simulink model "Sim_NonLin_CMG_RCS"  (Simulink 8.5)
settings: Solver=ode45  StartTime=0.0  StopTime=3600  FixedStep=Ts*2  RelTol=1e-3
InitFcn:
  | start3
StopFcn:
  | Pl
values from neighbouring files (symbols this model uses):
  Ave = [    [vehicle_flex34.m]    (also in vehicle_rigid.m)
  Bve = [    [vehicle_flex34.m]    (also in vehicle_rigid.m)
  CB2L = [cpsi, -cphi*spsi,  sphi*spsi;          0,    cphi,      -sphi;          0,    sphi*cpsi,  cphi*cpsi]/cpsi    [Rigbod_Dynam_LVLH.m]    (also in start.m = eye(3); start2.m = eye(3); start3.m = eye(3); start1.m = eye(3))
  com_dir = com_dir/sqrt(com_dir'*com_dir)    [start.m]    (also in start2.m; start3.m; start1.m)
  Cve = [    [vehicle_flex34.m]    (also in vehicle_rigid.m)
  d2r = pi/180    (= 0.0174532925199)    [start.m]    (also in start2.m; start3.m; Dead_Band_DF.m; start1.m)
  Dve = [    [vehicle_flex34.m]    (also in vehicle_rigid.m)
  ini = [wbo; atto; Hco]    [start.m]    (also in start2.m; start3.m; start1.m)
  J = [0.119416e9, -0.476e7,   -0.1216e7;     -0.476e7,     0.40408e8, -0.30121e6;     -0.1216e7,   -0.30121e6,  0.110166e9]    [start.m]    (also in start2.m; start3.m; start1.m)
  KshC = 2*Wdot_Lim_CMG/WlimC    [start.m]    (also in start2.m; start3.m; start1.m)
  KshR = 2*Wdot_Lim_RCS/WlimR    [start.m]    (also in start2.m; start3.m; start1.m)
  nt = 12    [start.m]    (also in start2.m; start3.m; start1.m)
  omg = 20*wo    (= 0.022)    [start.m]    (also in start2.m; start3.m; start1.m)
  r2d = 180/pi    (= 57.2957795131)    [start.m]    (also in start2.m; start3.m; start1.m)
  thecmd = 20    [start.m]    (also in start2.m; start3.m; start1.m = 0.1)
  Wdot_Lim_CMG = 0.0001*d2r    (= 1.74532925199e-06)    [start.m]    (also in start2.m; start3.m; start1.m)
  Wdot_Lim_RCS = 0.02*d2r    (= 0.000349065850399)    [start.m]    (also in start2.m; start3.m; start1.m)
  Wlim_CMG = 0.01*d2r    (= 0.000174532925199)    [start.m]    (also in start2.m; start3.m; start1.m)
  Wlim_RCS = 0.6*d2r    (= 0.010471975512)    [start.m]    (also in start2.m; start3.m; start1.m)
  wo = 0.0011    [start.m]    (also in start2.m; start3.m; start1.m)
  zeb = 0.95    [start.m]    (also in start2.m; start3.m; start1.m)
undefined symbols (not defined in the file or in its folder): Phase_Plane, Rigbod_Dynam_LVLH, Torq_Lim, Wlim

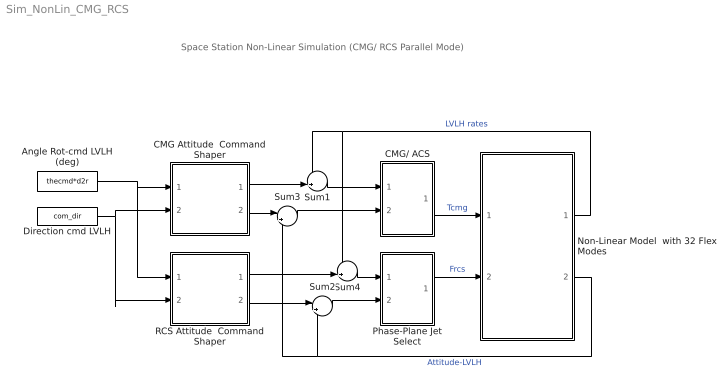
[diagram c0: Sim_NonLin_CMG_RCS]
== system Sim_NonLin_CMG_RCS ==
  note: Space Station Non-Linear Simulation (CMG/ RCS Parallel Mode)
  Angle Rot-cmd LVLH (deg) : Constant  Value=thecmd*d2r
  CMG Attitude  Command Shaper : Subsystem
  CMG/ ACS : Subsystem
  Direction cmd LVLH : Constant  Value=com_dir
  Non-Linear Model  with 32 Flex Modes : Subsystem
  Phase-Plane Jet Select : Subsystem
  RCS Attitude  Command Shaper : Subsystem
  Sum1 : Sum  Inputs=-+|
  Sum2 : Sum  Inputs=|+-
  Sum3 : Sum  Inputs=|+-
  Sum4 : Sum  Inputs=-+|
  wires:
  Non-Linear Model  with 32 Flex Modes/2(atti-lv) -> Sum2/2, Sum3/2  "Attitude-LVLH"
  Sum2/1 -> Phase-Plane Jet Select/2(atter)
  Non-Linear Model  with 32 Flex Modes/1(w-lv) -> Sum1/1, Sum4/1  "LVLH rates"
  Direction cmd LVLH/1 -> CMG Attitude  Command Shaper/2(dir), RCS Attitude  Command Shaper/2(dir)
  Angle Rot-cmd LVLH (deg)/1 -> RCS Attitude  Command Shaper/1(cmd), CMG Attitude  Command Shaper/1(cmd)
  Sum1/1 -> CMG/ ACS/1(wl)
  Sum3/1 -> CMG/ ACS/2(ater)
  RCS Attitude  Command Shaper/2(att-cmd) -> Sum2/1
  Phase-Plane Jet Select/1(f(i)) -> Non-Linear Model  with 32 Flex Modes/2(Frcs)  "Frcs"
  CMG/ ACS/1(Tq) -> Non-Linear Model  with 32 Flex Modes/1(Tcmg)  "Tcmg"
  Sum4/1 -> Phase-Plane Jet Select/1(rater)
  RCS Attitude  Command Shaper/1(w-cmd) -> Sum4/2
  CMG Attitude  Command Shaper/1(w-cmd) -> Sum1/2
  CMG Attitude  Command Shaper/2(att-cmd) -> Sum3/1

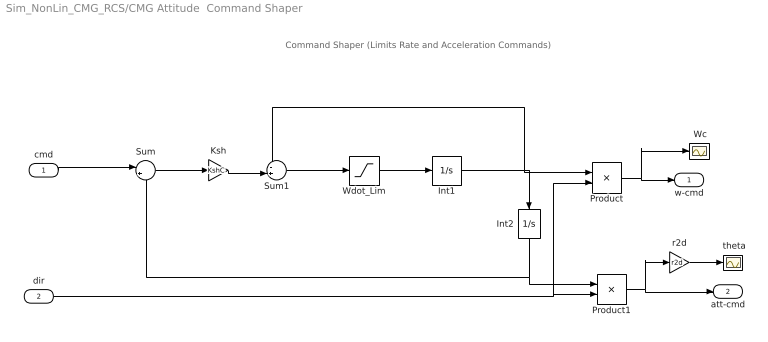
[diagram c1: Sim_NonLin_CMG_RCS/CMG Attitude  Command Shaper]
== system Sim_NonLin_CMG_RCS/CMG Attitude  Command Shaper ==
  note: Command Shaper (Limits Rate and Acceleration Commands)
  cmd : Inport  PortDimensions=1
  dir : Inport  Port=2  PortDimensions=3
  " Wc" : Scope
  " theta" : Scope
  Int1 : Integrator  LimitOutput=on  UpperSaturationLimit=Wlim_CMG  LowerSaturationLimit=-Wlim_CMG
  Int2 : Integrator  UpperSaturationLimit=Wlim  LowerSaturationLimit=-Wlim
  Ksh : Gain  Gain=KshC
  Product : Product
  Product1 : Product
  Sum : Sum  Inputs=|+-
  Sum1 : Sum  Inputs=-+|
  Wdot_Lim : Saturate  UpperLimit=Wdot_Lim_CMG  LowerLimit=-Wdot_Lim_CMG
  r2d : Gain  Gain=r2d
  w-cmd : Outport  PortDimensions=3
  att-cmd : Outport  Port=2  PortDimensions=3
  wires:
  Wdot_Lim/1 -> Int1/1
  Sum1/1 -> Wdot_Lim/1
  Int1/1 -> Product/1, Sum1/1, Int2/1
  Sum/1 -> Ksh/1
  Ksh/1 -> Sum1/2
  Int2/1 -> Sum/2, Product1/1
  cmd/1 -> Sum/1
  dir/1 -> Product/2, Product1/2
  r2d/1 -> " theta"/1
  Product/1 -> w-cmd/1, " Wc"/1
  Product1/1 -> att-cmd/1, r2d/1

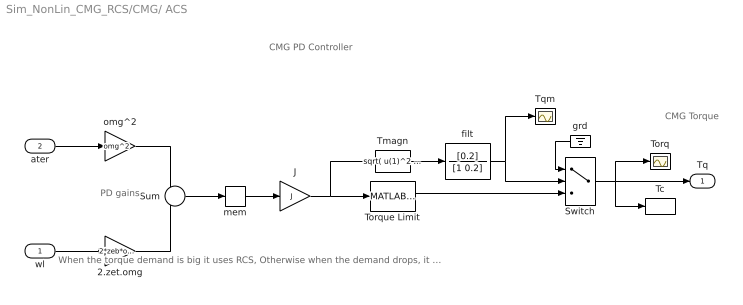
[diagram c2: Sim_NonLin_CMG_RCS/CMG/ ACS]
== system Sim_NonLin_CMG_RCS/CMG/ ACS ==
  note: CMG PD Controller
  note: PD gains
  note: CMG Torque
  note: When the torque demand is big it uses RCS, Otherwise when the demand drops, it switches to CMG Control to avoid Saturating the CMGs
  wl : Inport
  ater : Inport  Port=2  PortDimensions=3
  2.zet.omg : Gain  Gain=2*zeb*omg
  J : Gain  Gain=J  Multiplication=Matrix(K*u)
  Sum : Sum  Inputs=--
  Switch : Switch  Threshold=2500
  Tc : ToWorkspace  VariableName=Tcmg  SampleTime=-1
  Tmagn : Fcn  Expr=sqrt( u(1)^2 + u(2)^2 + u(3)^2 )
  Torq : Scope
  Torque Limit : MATLABFcn  MATLABFcn=Torq_Lim( u(1:3) )  OutputDimensions=3
  Tqm : Scope
  filt : TransferFcn  Numerator=[0.2]  Denominator=[1 0.2]
  grd : Ground
  mem : Memory
  omg^2 : Gain  Gain=omg^2
  Tq : Outport
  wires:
  wl/1 -> 2.zet.omg/1
  Sum/1 -> mem/1
  2.zet.omg/1 -> Sum/2
  ater/1 -> omg^2/1
  omg^2/1 -> Sum/1
  J/1 -> Torque Limit/1, Tmagn/1
  mem/1 -> J/1
  Torque Limit/1 -> Switch/3
  Switch/1 -> Tq/1, Torq/1, Tc/1
  Tmagn/1 -> filt/1
  grd/1 -> Switch/1
  filt/1 -> Switch/2, Tqm/1

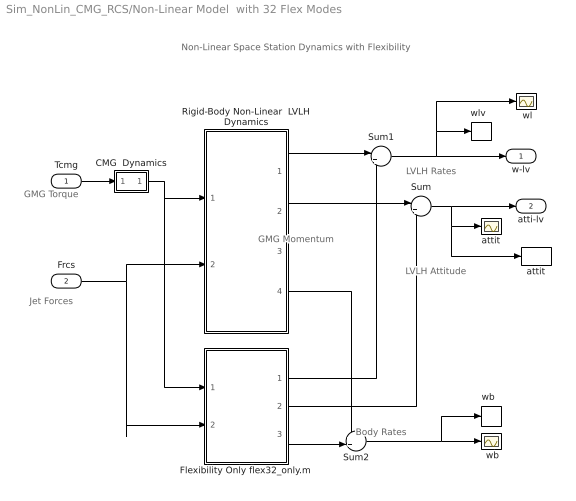
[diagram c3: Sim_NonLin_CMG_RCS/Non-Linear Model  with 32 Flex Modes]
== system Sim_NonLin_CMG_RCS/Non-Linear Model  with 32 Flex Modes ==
  note: LVLH Rates
  note: Non-Linear Space Station Dynamics with Flexibility
  note: LVLH Attitude
  note: Body Rates
  note: GMG Torque
  note: Jet Forces
  note: GMG Momentum
  Tcmg : Inport
  Frcs : Inport  Port=2
  " attit " : Scope
  " wb" : Scope
  " wl" : Scope
  CMG  Dynamics : Subsystem
  Flexibility Only flex32_only.m : Subsystem
  Rigid-Body Non-Linear  LVLH Dynamics : Subsystem
  Sum : Sum  Inputs=|++
  Sum1 : Sum  Inputs=|++
  Sum2 : Sum  Inputs=++|
  attit : ToWorkspace  VariableName=theta  SampleTime=-1
  "wb  " : ToWorkspace  VariableName=wb  SampleTime=-1
  "wlv  " : ToWorkspace  VariableName=wl  SampleTime=-1
  w-lv : Outport
  atti-lv : Outport  Port=2
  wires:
  Frcs/1 -> Rigid-Body Non-Linear  LVLH Dynamics/2(Frcs), Flexibility Only flex32_only.m/2(Frcs)
  Rigid-Body Non-Linear  LVLH Dynamics/2(atti-lv) -> Sum/1
  Flexibility Only flex32_only.m/2(att) -> Sum/2
  Sum/1 -> atti-lv/1, " attit "/1, attit/1
  Sum1/1 -> w-lv/1, "wlv  "/1, " wl"/1
  Tcmg/1 -> CMG  Dynamics/1(I)
  Rigid-Body Non-Linear  LVLH Dynamics/1(w-lv) -> Sum1/1
  Flexibility Only flex32_only.m/1(wlf) -> Sum1/2
  Flexibility Only flex32_only.m/3(wb) -> Sum2/2
  Rigid-Body Non-Linear  LVLH Dynamics/4(wb) -> Sum2/1
  Sum2/1 -> " wb"/1, "wb  "/1
  CMG  Dynamics/1(O) -> Rigid-Body Non-Linear  LVLH Dynamics/1(Tcmg), Flexibility Only flex32_only.m/1(Tcmg)

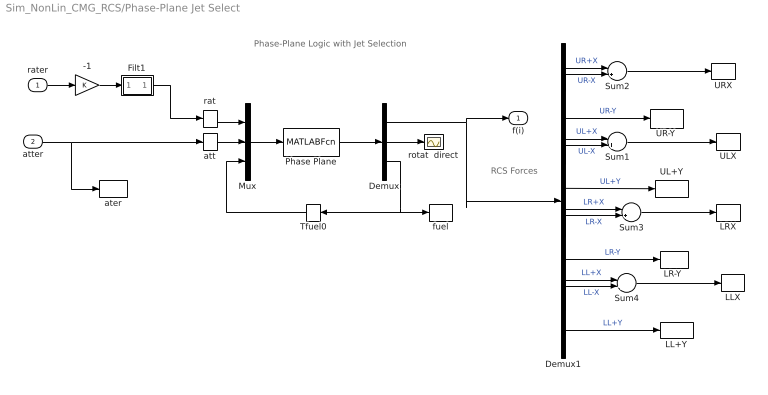
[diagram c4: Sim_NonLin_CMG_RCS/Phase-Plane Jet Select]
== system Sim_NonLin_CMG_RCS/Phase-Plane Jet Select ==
  note: Phase-Plane Logic with Jet Selection
  note: RCS Forces
  rater : Inport
  atter : Inport  Port=2
  -1 : Gain
  Demux : Demux  Outputs=[nt, 3,1]
  Demux1 : Demux  Outputs=nt
  Filt1 : Subsystem
  LL+Y : ToWorkspace  VariableName=LLPY  SampleTime=-1
  LLX : ToWorkspace  VariableName=LLX  SampleTime=-1
  "LR-Y " : ToWorkspace  VariableName=LRNY  SampleTime=-1
  LRX : ToWorkspace  VariableName=LRX  SampleTime=-1
  Mux : Mux  Inputs="[3  3  1]"
  Phase Plane : MATLABFcn  MATLABFcn=Phase_Plane( u(1:3), u(4:6), u(7) )  OutputDimensions=nt + 4
  Sum{1..4} (4 alike) : Sum  Inputs=|++
  Tfuel0 : Memory
  UL+Y : ToWorkspace  VariableName=ULPY  SampleTime=-1
  ULX : ToWorkspace  VariableName=ULX  SampleTime=-1
  "UR-Y " : ToWorkspace  VariableName=URNY  SampleTime=-1
  URX : ToWorkspace  VariableName=URX  SampleTime=-1
  ater : ToWorkspace  VariableName=atter  SampleTime=-1
  att : Memory
  fuel : ToWorkspace  VariableName=Fuel  SampleTime=-1
  rat : Memory
  rotat  direct : Scope
  f(i) : Outport
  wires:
  Demux/3 -> Tfuel0/1, fuel/1
  att/1 -> Mux/2
  atter/1 -> ater/1, att/1
  rater/1 -> -1/1
  Demux/2 -> rotat  direct/1
  Demux/1 -> f(i)/1, Demux1/1
  Tfuel0/1 -> Mux/3
  Phase Plane/1 -> Demux/1
  Mux/1 -> Phase Plane/1
  rat/1 -> Mux/1
  Demux1/1 -> Sum2/1  "UR+X"
  Demux1/2 -> Sum2/2  "UR-X"
  Sum2/1 -> URX/1
  Demux1/4 -> Sum1/1  "UL+X"
  Demux1/5 -> Sum1/2  "UL-X"
  Demux1/7 -> Sum3/1  "LR+X"
  Demux1/8 -> Sum3/2  "LR-X"
  Demux1/10 -> Sum4/1  "LL+X"
  Demux1/11 -> Sum4/2  "LL-X"
  Sum1/1 -> ULX/1
  Sum3/1 -> LRX/1
  Sum4/1 -> LLX/1
  Demux1/3 -> "UR-Y "/1  "UR-Y"
  Demux1/6 -> UL+Y/1  "UL+Y"
  Demux1/12 -> LL+Y/1  "LL+Y"
  Demux1/9 -> "LR-Y "/1  "LR-Y"
  -1/1 -> Filt1/1(I)
  Filt1/1(O) -> rat/1

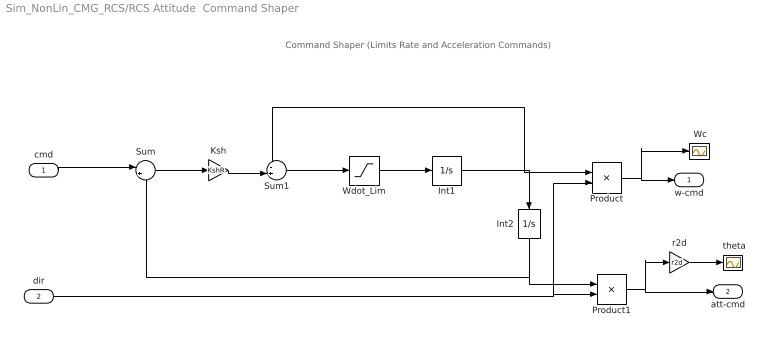
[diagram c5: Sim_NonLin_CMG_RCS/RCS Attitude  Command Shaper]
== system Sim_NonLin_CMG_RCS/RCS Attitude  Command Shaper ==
  note: Command Shaper (Limits Rate and Acceleration Commands)
  cmd : Inport  PortDimensions=1
  dir : Inport  Port=2  PortDimensions=3
  " Wc" : Scope
  " theta" : Scope
  Int1 : Integrator  LimitOutput=on  UpperSaturationLimit=Wlim_RCS  LowerSaturationLimit=-Wlim_RCS
  Int2 : Integrator  UpperSaturationLimit=Wlim  LowerSaturationLimit=-Wlim
  Ksh : Gain  Gain=KshR
  Product : Product
  Product1 : Product
  Sum : Sum  Inputs=|+-
  Sum1 : Sum  Inputs=-+|
  Wdot_Lim : Saturate  UpperLimit=Wdot_Lim_RCS  LowerLimit=-Wdot_Lim_RCS
  r2d : Gain  Gain=r2d
  w-cmd : Outport  PortDimensions=3
  att-cmd : Outport  Port=2  PortDimensions=3
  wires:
  Wdot_Lim/1 -> Int1/1
  Sum1/1 -> Wdot_Lim/1
  Int1/1 -> Product/1, Sum1/1, Int2/1
  Sum/1 -> Ksh/1
  Ksh/1 -> Sum1/2
  Int2/1 -> Sum/2, Product1/1
  cmd/1 -> Sum/1
  dir/1 -> Product/2, Product1/2
  r2d/1 -> " theta"/1
  Product/1 -> w-cmd/1, " Wc"/1
  Product1/1 -> att-cmd/1, r2d/1

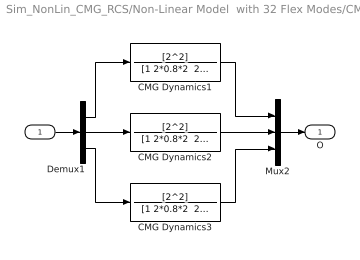
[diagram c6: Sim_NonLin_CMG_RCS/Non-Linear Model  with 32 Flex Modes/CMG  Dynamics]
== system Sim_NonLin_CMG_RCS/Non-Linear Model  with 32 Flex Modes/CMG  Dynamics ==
  I : Inport
  CMG Dynamics1 : TransferFcn  Numerator=[2^2]  Denominator="[1 2*0.8*2  2^2]"
  CMG Dynamics2 : TransferFcn  Numerator=[2^2]  Denominator="[1 2*0.8*2  2^2]"
  CMG Dynamics3 : TransferFcn  Numerator=[2^2]  Denominator="[1 2*0.8*2  2^2]"
  Demux1 : Demux  Outputs=3
  Mux2 : Mux  Inputs=3
  O : Outport
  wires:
  Mux2/1 -> O/1
  I/1 -> Demux1/1
  Demux1/3 -> CMG Dynamics3/1
  Demux1/1 -> CMG Dynamics1/1
  Demux1/2 -> CMG Dynamics2/1
  CMG Dynamics1/1 -> Mux2/1
  CMG Dynamics3/1 -> Mux2/3
  CMG Dynamics2/1 -> Mux2/2

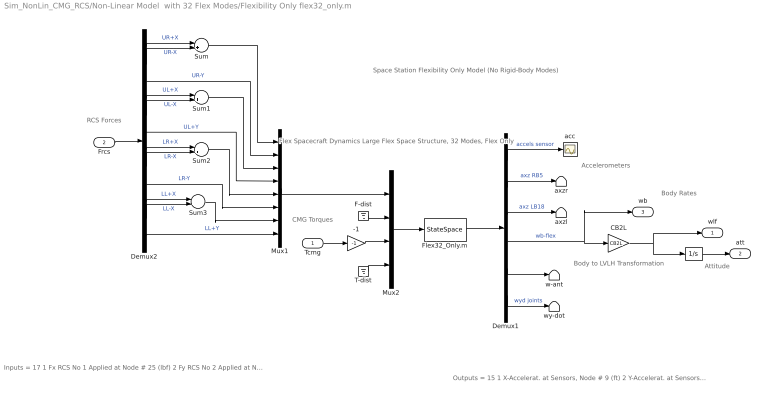
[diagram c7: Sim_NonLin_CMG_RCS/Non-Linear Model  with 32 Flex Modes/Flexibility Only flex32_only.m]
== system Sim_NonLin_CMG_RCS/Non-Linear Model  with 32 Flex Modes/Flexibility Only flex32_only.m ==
  note: Outputs = 15 1 X-Accelerat. at Sensors, Node # 9 (ft) 2 Y-Accelerat. at Sensors, Node # 9 (ft) 3 Z-Accelerat. at Sensors, Node # 9 (ft) 4 X-Accelerat. at Right Boom End, Node # 5 (ft) 5 Z-Accelerat. at Right Boom End, Node # 5 (ft) 6 X-Accelerat. at Left Boom End, Node # 18 (ft) 7 Z-Accelerat. at Left Boom End, Node # 18 (ft) 8 X-Rot. Rate at Sensors, Node # 9 (radian) 9 Y-Rot. Rate at Sensors, Node # 9 (radian) 10 Z-Rot. Rate at Sensors, Node # 9 (radian) 11 X-Rot. Rate at Antena Bot-Left, Node # 24 (radian) 12 Y-Rot. Rate at Antena Bot-Left, Node # 24 (radian) 13 Z-Rot. Rate at Antena Bot-Left, Node # 24 (radian) 14 Y-Rot.Accel. at Right Joint, Node # 7 (radian) 15 Y-Rot.Accel. at Left Joint, Node # 16 (radian)
  note: Inputs = 17 1 Fx RCS No 1 Applied at Node # 25 (lbf) 2 Fy RCS No 2 Applied at Node # 25 (lbf) 3 Fx RCS No 3 Applied at Node # 26 (lbf) 4 Fy RCS No 4 Applied at Node # 26 (lbf) 5 Fx RCS No 5 Applied at Node # 27 (lbf) 6 Fy RCS No 6 Applied at Node # 27 (lbf) 7 Fx RCS No 7 Applied at Node # 28 (lbf) 8 Fy RCS No 8 Applied at Node # 28 (lbf) 9 Fx Disturb. No 9 at Node # 21 (lbf) 10 Fy Disturb. No 10 at Node # 21 (lbf) 11 Fz Disturb. No 11 at Node # 21 (lbf) 12 Torq-x No 1 CMG Applied at Node # 10 (ft-lb) 13 Torq-y No 2 CMG Applied at Node # 10 (ft-lb) 14 Torq-z No 3 CMG Applied at Node # 10 (ft-lb) 15 Torq-x No 4 Gimbal Dist. at Node # 1 (ft-lb) 16 Torq-y No 5 Gimbal Dist. at Node # 1 (ft-lb) 17 Torq-z No 6 Gimbal Dist. at Node # 1 (ft-lb)
  note: Space Station Flexibility Only Model (No Rigid-Body Modes)
  note: Body to LVLH Transformation
  note: RCS Forces
  note: Flex Spacecraft Dynamics Large Flex Space Structure, 32 Modes, Flex Only
  note: Accelerometers
  note: Body Rates
  note: Attitude
  note: CMG Torques
  Tcmg : Inport
  Frcs : Inport  Port=2
  "  " : Integrator
  -1 : Gain  Gain=-1
  CB2L : Gain  Gain=CB2L  Multiplication=Matrix(K*u)
  Demux1 : Demux  Outputs=[3, 2, 2, 3, 3, 2]
  Demux2 : Demux  Outputs=12
  F-dist : Ground
  Flex32_Only.m : StateSpace  A=Ave  B=Bve  C=Cve  D=Dve  X0=0
  Mux1 : Mux  Inputs=8
  Mux2 : Mux  Inputs=[8, 3, 3, 3]
  Sum{,1..3} (4 alike) : Sum  Inputs=|+-
  T-dist : Ground
  acc : Scope
  axzl : Terminator
  axzr : Terminator
  w-ant : Terminator
  wy-dot : Terminator
  wlf : Outport
  att : Outport  Port=2
  wb : Outport  Port=3
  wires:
  Demux1/6 -> wy-dot/1  "wyd joints"
  Demux1/5 -> w-ant/1
  T-dist/1 -> Mux2/4
  F-dist/1 -> Mux2/2
  Demux1/3 -> axzl/1  "axz LB18"
  Demux1/2 -> axzr/1  "axz RB5"
  Tcmg/1 -> -1/1
  Demux1/4 -> CB2L/1, wb/1  "wb-flex"
  Demux1/1 -> acc/1  "accels sensor"
  Flex32_Only.m/1 -> Demux1/1
  Mux2/1 -> Flex32_Only.m/1
  Mux1/1 -> Mux2/1
  Frcs/1 -> Demux2/1
  Demux2/6 -> Mux1/4  "UL+Y"
  Demux2/9 -> Mux1/6  "LR-Y"
  Demux2/12 -> Mux1/8  "LL+Y"
  Demux2/3 -> Mux1/2  "UR-Y"
  Demux2/1 -> Sum/1  "UR+X"
  Demux2/2 -> Sum/2  "UR-X"
  Sum/1 -> Mux1/1
  Demux2/4 -> Sum1/1  "UL+X"
  Demux2/5 -> Sum1/2  "UL-X"
  Sum1/1 -> Mux1/3
  Demux2/7 -> Sum2/1  "LR+X"
  Demux2/8 -> Sum2/2  "LR-X"
  Demux2/10 -> Sum3/1  "LL+X"
  Demux2/11 -> Sum3/2  "LL-X"
  Sum3/1 -> Mux1/7
  Sum2/1 -> Mux1/5
  "  "/1 -> att/1
  -1/1 -> Mux2/3
  CB2L/1 -> wlf/1, "  "/1

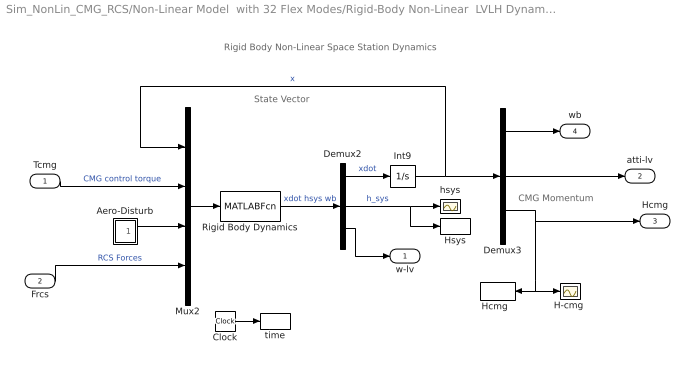
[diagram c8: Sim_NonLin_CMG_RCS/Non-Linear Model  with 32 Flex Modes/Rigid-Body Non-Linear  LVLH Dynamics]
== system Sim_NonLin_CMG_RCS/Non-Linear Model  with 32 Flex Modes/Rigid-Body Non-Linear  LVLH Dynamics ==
  note: CMG Momentum
  note: State Vector
  note: Rigid Body Non-Linear Space Station Dynamics
  Tcmg : Inport  PortDimensions=3
  Frcs : Inport  Port=2  PortDimensions=nt
  Aero-Disturb : Subsystem
  Clock : Clock
  Demux2 : Demux  Outputs=[9,3,3]
  Demux3 : Demux  Outputs=[3,3,3]
  "H-cmg " : Scope
  "Hcmg  " : ToWorkspace  VariableName=Hcmg  SampleTime=-1
  Hsys : ToWorkspace  VariableName=Hsys  SampleTime=-1
  Int9 : Integrator  InitialCondition=ini
  Mux2 : Mux  Inputs=[9, 3, 3, nt]
  Rigid Body Dynamics : MATLABFcn  MATLABFcn=Rigbod_Dynam_LVLH( u(1:9), u(10:12), u(13:15), u(16:15+nt) )  OutputDimensions=15
  hsys : Scope
  time : ToWorkspace  VariableName=time  SampleTime=-1
  w-lv : Outport
  atti-lv : Outport  Port=2
  Hcmg : Outport  Port=3
  wb : Outport  Port=4
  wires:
  Mux2/1 -> Rigid Body Dynamics/1
  Clock/1 -> time/1
  Frcs/1 -> Mux2/4  "RCS Forces"
  Demux3/3 -> Hcmg/1, "H-cmg "/1, "Hcmg  "/1
  Demux3/2 -> atti-lv/1
  Demux2/2 -> Hsys/1, hsys/1  "h_sys"
  Demux2/3 -> w-lv/1
  Tcmg/1 -> Mux2/2  "CMG control torque"
  Int9/1 -> Mux2/1, Demux3/1  "x"
  Demux2/1 -> Int9/1  "xdot"
  Rigid Body Dynamics/1 -> Demux2/1  "xdot hsys wb"
  Aero-Disturb/1(Td) -> Mux2/3
  Demux3/1 -> wb/1

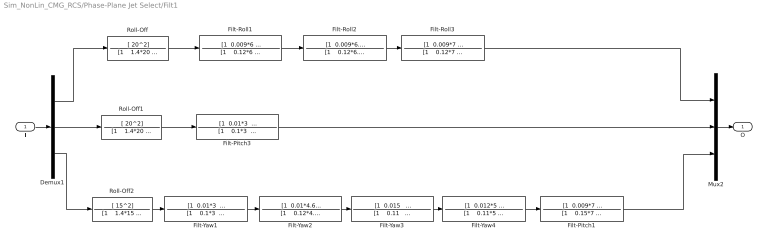
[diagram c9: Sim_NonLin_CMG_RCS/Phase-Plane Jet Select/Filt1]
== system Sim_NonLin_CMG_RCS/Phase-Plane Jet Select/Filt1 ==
  I : Inport
  Demux1 : Demux  Outputs=3
  Filt-Pitch1 : TransferFcn  Numerator="[1  0.009*7   6.83^2]"  Denominator="[1    0.15*7    6.83^2]"
  Filt-Pitch3 : TransferFcn  Numerator="[1  0.01*3   3.07^2]"  Denominator="[1    0.1*3    3.07^2]"
  Filt-Roll1 : TransferFcn  Numerator="[1  0.009*6   5.85^2]"  Denominator="[1    0.12*6    5.85^2]"
  Filt-Roll2 : TransferFcn  Numerator="[1  0.009*6.4   6.46^2]"  Denominator="[1    0.12*6.4    6.46^2]"
  Filt-Roll3 : TransferFcn  Numerator="[1  0.009*7   7.51^2]"  Denominator="[1    0.12*7    7.51^2]"
  Filt-Yaw1 : TransferFcn  Numerator="[1  0.01*3   3.07^2]"  Denominator="[1    0.1*3    3.07^2]"
  Filt-Yaw2 : TransferFcn  Numerator="[1  0.01*4.6   4.6^2]"  Denominator="[1    0.12*4.6    4.6^2]"
  Filt-Yaw3 : TransferFcn  Numerator="[1  0.015   1.14^2]"  Denominator="[1    0.11    1.14^2]"
  Filt-Yaw4 : TransferFcn  Numerator="[1  0.012*5   5.21^2]"  Denominator="[1    0.11*5    5.21^2]"
  Mux2 : Mux  Inputs=3
  Roll-Off : TransferFcn  Numerator=[ 20^2]  Denominator="[1    1.4*20    20^2]"
  Roll-Off1 : TransferFcn  Numerator=[ 20^2]  Denominator="[1    1.4*20    20^2]"
  Roll-Off2 : TransferFcn  Numerator=[ 15^2]  Denominator="[1    1.4*15    15^2]"
  O : Outport
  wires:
  I/1 -> Demux1/1
  Mux2/1 -> O/1
  Demux1/1 -> Roll-Off/1
  Demux1/3 -> Roll-Off2/1
  Demux1/2 -> Roll-Off1/1
  Roll-Off/1 -> Filt-Roll1/1
  Roll-Off2/1 -> Filt-Yaw1/1
  Roll-Off1/1 -> Filt-Pitch3/1
  Filt-Roll1/1 -> Filt-Roll2/1
  Filt-Roll2/1 -> Filt-Roll3/1
  Filt-Roll3/1 -> Mux2/1
  Filt-Pitch3/1 -> Mux2/2
  Filt-Yaw1/1 -> Filt-Yaw2/1
  Filt-Yaw2/1 -> Filt-Yaw3/1
  Filt-Yaw3/1 -> Filt-Yaw4/1
  Filt-Yaw4/1 -> Filt-Pitch1/1
  Filt-Pitch1/1 -> Mux2/3

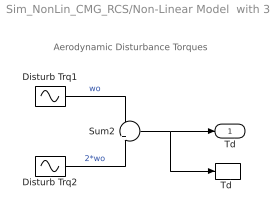
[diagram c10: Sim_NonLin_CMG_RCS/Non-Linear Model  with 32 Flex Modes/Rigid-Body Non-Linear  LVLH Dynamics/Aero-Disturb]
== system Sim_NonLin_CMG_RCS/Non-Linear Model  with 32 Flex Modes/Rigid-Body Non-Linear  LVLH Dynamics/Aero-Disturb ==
  note: Aerodynamic Disturbance Torques
  Disturb Trq1 : Sin  Amplitude=[1, 3, 1]  Bias="[1  8  1]"  Frequency=[wo, wo, wo]  SampleTime=0
  Disturb Trq2 : Sin  Amplitude=[1, 1, 1]*0.5  Frequency=[wo, wo, wo]*2  SampleTime=0
  Sum2 : Sum  Inputs=+|+
  "Td " : ToWorkspace  VariableName=Td  SampleTime=-1
  Td : Outport
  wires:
  Disturb Trq2/1 -> Sum2/2  "2*wo"
  Sum2/1 -> "Td "/1, Td/1
  Disturb Trq1/1 -> Sum2/1  "wo"
